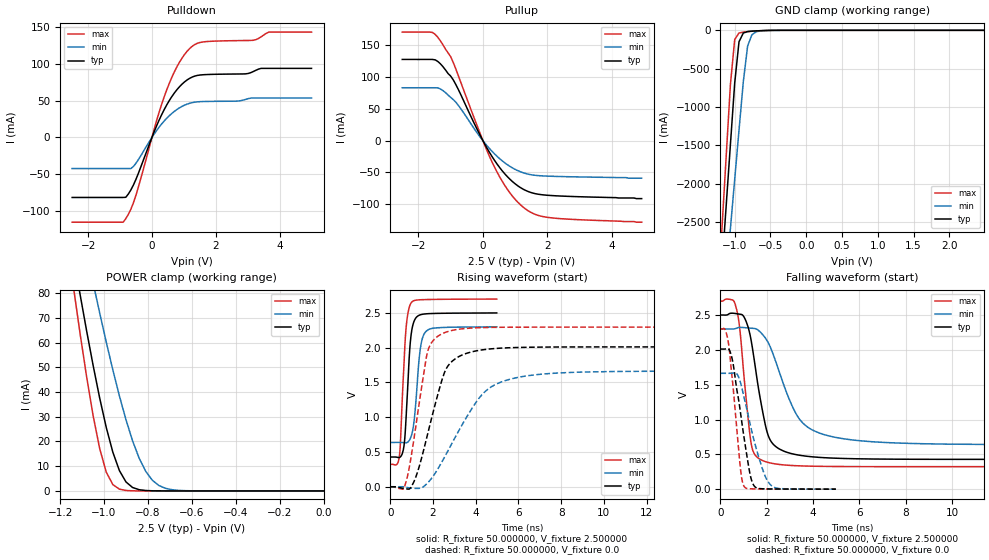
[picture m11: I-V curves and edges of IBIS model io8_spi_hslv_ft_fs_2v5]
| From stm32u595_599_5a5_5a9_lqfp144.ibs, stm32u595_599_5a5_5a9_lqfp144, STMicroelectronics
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|   Model io8_spi_hslv_ft_fs_2v5
[Model]  io8_spi_hslv_ft_fs_2v5
Model_type I/O
Polarity   Non-Inverting
Enable   Active-Low
Vinl =   0.750000V
Vinh =   1.750000V
Vmeas =  1.250000V
Cref =   50.000000pF
Rref =   100.000000M
Vref =   0.0V
C_comp   3.438200pF   3.436700pF   3.473300pF
[Temperature Range]   25.000000   0.140000k   -40.000000
[Pullup Reference]   2.500000V   2.300000V   2.700000V
[Pulldown Reference]   0.0V   0.0V   0.0V
[POWER Clamp Reference]   2.500000V   2.300000V   2.700000V
[GND Clamp Reference]   0.0V   0.0V   0.0V
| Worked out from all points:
|   slope of the pulldown table from 0 to 0.375 V, typ, clamps not added: 10.1 ohm
|   slope of the pullup table from 0 to 0.375 V, typ, clamps not added: 11.7 ohm
|   GND clamp passes 1 mA (typ) near -0.50 V on its own axis
|   POWER clamp passes 1 mA (typ) near -0.86 V on its own axis
|   rising waveform, R_fixture 50.000000, V_fixture 2.500000: 20-80 % time 229ps typ, 275ps min, 225ps max; typ from 0.428 V to 2.5 V
|   rising waveform, R_fixture 50.000000, V_fixture 0.0: 20-80 % time 1.04ns typ, 1.94ns min, 685ps max; typ from 0 V to 2.01 V
|   falling waveform, R_fixture 50.000000, V_fixture 2.500000: 20-80 % time 645ps typ, 1.26ns min, 407ps max; typ from 2.5 V to 0.428 V
|   falling waveform, R_fixture 50.000000, V_fixture 0.0: 20-80 % time 548ps typ, 765ps min, 383ps max; typ from 2.01 V to 0 V
[Pulldown]
|Voltage   I(typ)   I(min)   I(max)
-2.5V     -81.62mA   -42.31mA   -115.3mA
-900mV    -81.62mA   -42.31mA   -115.3mA
-820mV    -81.42mA   -42.31mA   -110.6mA
-500mV    -56.95mA   -35.08mA   -78.57mA
140mV     15.18mA    9.02mA     22.02mA
460mV     44mA       25.98mA    64.38mA
860mV     68.91mA    40.27mA    102.2mA
1.26V     82.21mA    47.42mA    124mA
1.66V     85.53mA    48.99mA    130.3mA
3.18V     89.84mA    53.65mA    132.3mA
3.66V     94.05mA    53.65mA    143.4mA
5V        94.05mA    53.65mA    143.4mA
[Pullup]
|Voltage   I(typ)   I(min)   I(max)
-2.5V     127.4mA    83mA       170.4mA
-1.56V    127.4mA    83mA       169.7mA
-1.32V    120.7mA    81.18mA    156.8mA
-1V       101.4mA    67.89mA    131.8mA
-920mV    95.46mA    64.48mA    122.7mA
-40mV     3.893mA    2.628mA    5.181mA
360mV     -30.97mA   -20.78mA   -41.56mA
760mV     -56.64mA   -37.85mA   -76.55mA
1.24V     -75.99mA   -50.28mA   -104.1mA
1.64V     -83.42mA   -54.54mA   -116.1mA
2.04V     -85.88mA   -55.77mA   -120.6mA
4.92V     -91mA      -59mA      -128mA
[GND_clamp]
|Voltage   I(typ)   I(min)   I(max)
-2.5V     -9.641A    -9.693A    -9.352A
-1.18V    -3.114A    -3.874A    -2.614A
-1.12V    -2.301A    -3.23A     -1.656A
-1.06V    -1.489A    -2.587A    -706.2mA
-1V       -685.8mA   -1.945A    -119.3mA
-940mV    -149.7mA   -1.304A    -34.73mA
-880mV    -35.54mA   -672.6mA   -23.06mA
-820mV    -16.19mA   -206.4mA   -17.27mA
-760mV    -10.58mA   -57.55mA   -12.41mA
-700mV    -7.152mA   -18.74mA   -8.24mA
-400mV    -103.3uA   -378.5uA   -41.74uA
2.48V     0A         13.22nA    0A
[POWER_clamp]
|Voltage   I(typ)   I(min)   I(max)
-2.49V    881mA      773.1mA    1.07A
-1.14V    95.25mA    122.7mA    82.82mA
-1.11V    79.9mA     109.7mA    64.14mA
-1.05V    50.87mA    84.26mA    30.57mA
-1.02V    37.63mA    72.04mA    17.17mA
-990mV    25.71mA    60.25mA    7.621mA
-930mV    8.217mA    38.43mA    713.9uA
-900mV    3.624mA    28.77mA    182.8uA
-840mV    490.7uA    13.24mA    11.35uA
-780mV    56.55uA    4.324mA    699nA
-660mV    716.7nA    226uA      9.786nA
0V        0A         19.53nA    0A
[Ramp]
| variable   typ   min   max
dV/dt_r  1.20666/1.04148n   0.99780/1.94066n   1.37784/0.68377n
dV/dt_f  1.24344/0.64467n   0.99742/1.25468n   1.42636/0.40595n
R_load = 50.000000
[Rising Waveform]
R_fixture= 50.000000
V_fixture= 2.500000
V_fixture_min= 2.300000
V_fixture_max= 2.700000
|time   V(typ)   V(min)   V(max)
0s        427.6mV    637.6mV    322.8mV
420.4ps   421.2mV    637.6mV    425.2mV
470.5ps   429.1mV    637.6mV    607.3mV
640.6ps   582.7mV    633.8mV    1.753V
770.8ps   1.169V     634.7mV    2.376V
971ps     2.172V     721.4mV    2.642V
1.121ns   2.386V     962.6mV    2.678V
1.401ns   2.472V     1.973V     2.689V
1.622ns   2.485V     2.216V     2.692V
4.985ns   2.5V       2.3V       2.7V
[Rising Waveform]
R_fixture= 50.000000
V_fixture= 0.0
V_fixture_min= 0.0
V_fixture_max= 0.0
|time   V(typ)   V(min)   V(max)
0s        -32.77uV   -5.735uV   52.51uV
640.6ps   -24.21mV   -1.11mV    -17.07mV
840.8ps   -34.45mV   -13.74mV   201.8mV
1.081ns   55.67mV    -21.74mV   633.3mV
1.762ns   773.1mV    58.99mV    1.958V
2.563ns   1.66V      438.3mV    2.218V
3.123ns   1.857V     758.7mV    2.262V
4.284ns   1.968V     1.321V     2.289V
5.846ns   2.002V     1.565V     2.295V
19.94ns   2.011V     1.663V     2.296V
[Falling Waveform]
R_fixture= 50.000000
V_fixture= 2.500000
V_fixture_min= 2.300000
V_fixture_max= 2.700000
|time   V(typ)   V(min)   V(max)
0s        2.5V       2.3V       2.7V
680.7ps   2.52V      2.308V     2.606V
840.8ps   2.512V     2.322V     2.292V
1.121ns   2.399V     2.317V     1.266V
1.401ns   1.987V     2.309V     554.2mV
1.922ns   950.6mV    2.179V     397.9mV
2.322ns   631.2mV    1.895V     365.2mV
3.403ns   487.8mV    1.01V      334.8mV
4.685ns   448.5mV    764.5mV    326.3mV
19.94ns   427.6mV    637.6mV    322.8mV
[Falling Waveform]
R_fixture= 50.000000
V_fixture= 0.0
V_fixture_min= 0.0
V_fixture_max= 0.0
|time   V(typ)   V(min)   V(max)
0s        2.011V     1.663V     2.296V
190.2ps   2.011V     1.663V     2.294V
340.3ps   2.017V     1.663V     2.112V
530.5ps   1.834V     1.666V     1.523V
870.9ps   1.09V      1.525V     279.6mV
1.041ns   697.6mV    1.287V     31.17mV
1.421ns   66.15mV    741.3mV    4.24mV
1.892ns   4.942mV    220.4mV    2.165mV
2.182ns   2.989mV    57.17mV    1.689mV
4.985ns   -32.77uV   -5.735uV   52.51uV
